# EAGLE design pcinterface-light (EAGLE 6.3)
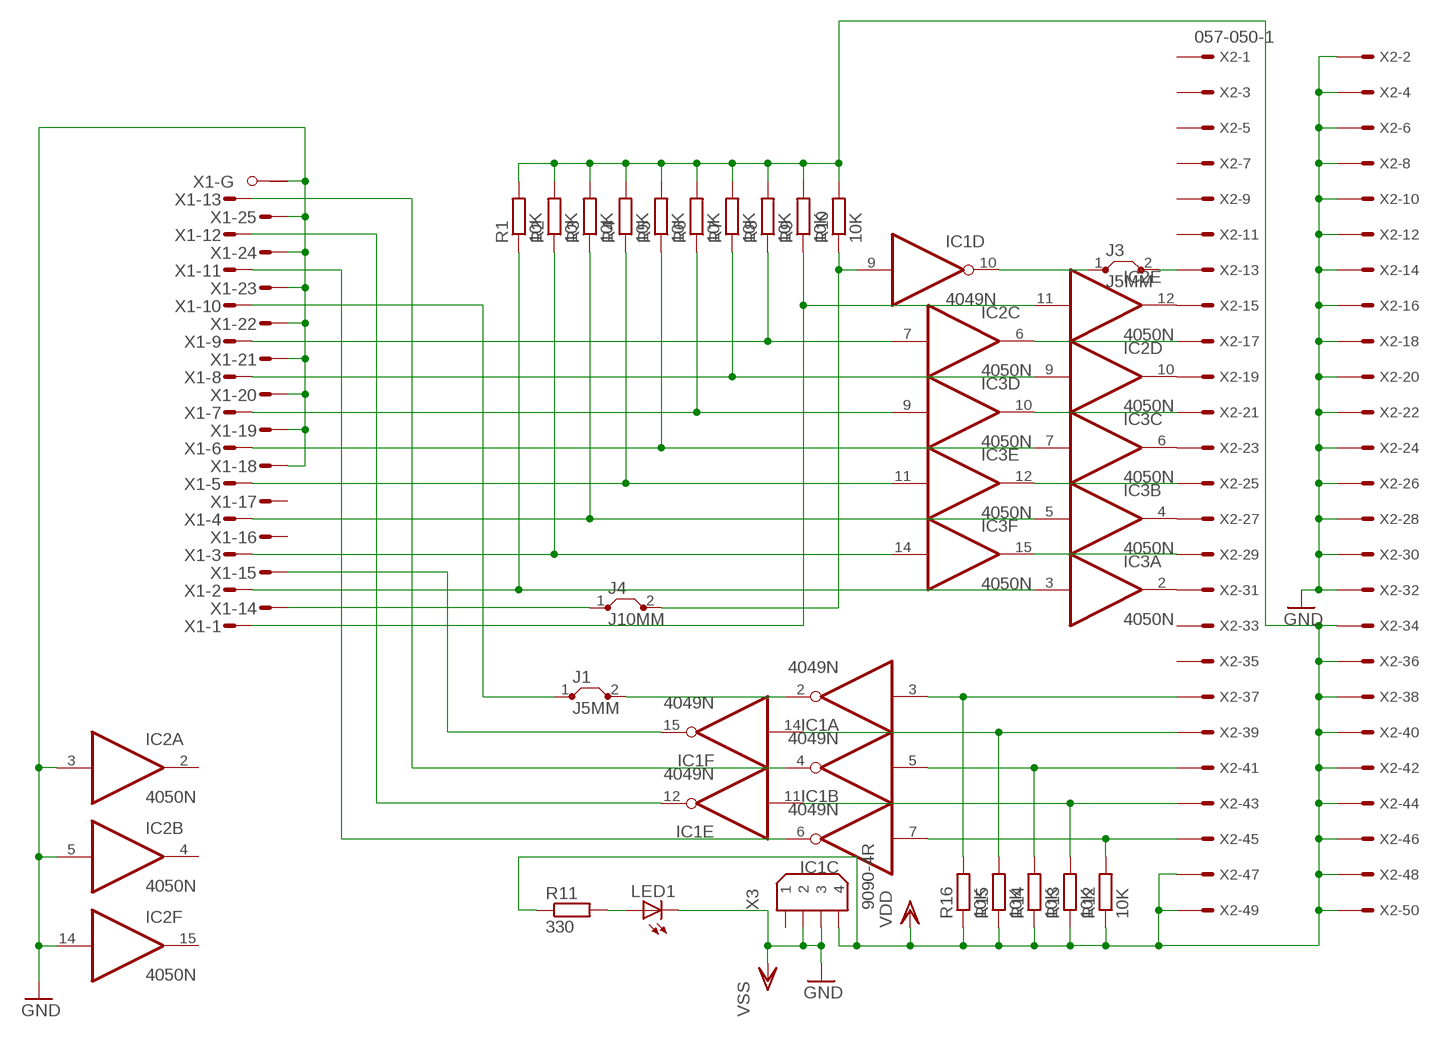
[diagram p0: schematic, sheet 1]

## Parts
IC1  4049N  [DIL16]
IC2  4050N  [DIL16]
IC3  4050N  [DIL16]
J1  J5MM  [05]
J3  J5MM  [05]
J4  J10MM  [10]
LED1  LED3MM  [LED3MM]
R1  10K  R-EU_0207/10  [0207/10]
R2  10K  R-EU_0207/10  [0207/10]
R3  10K  R-EU_0207/10  [0207/10]
R4  10K  R-EU_0207/10  [0207/10]
R5  10K  R-EU_0207/10  [0207/10]
R6  10K  R-EU_0207/10  [0207/10]
R7  10K  R-EU_0207/10  [0207/10]
R8  10K  R-EU_0207/10  [0207/10]
R9  10K  R-EU_0207/10  [0207/10]
R10  10K  R-EU_0207/10  [0207/10]
R11  330  R-EU_0207/10  [0207/10]
R12  10K  R-EU_0207/10  [0207/10]
R13  10K  R-EU_0207/10  [0207/10]
R14  10K  R-EU_0207/10  [0207/10]
R15  10K  R-EU_0207/10  [0207/10]
R16  10K  R-EU_0207/10  [0207/10]
X1  M25HPS  [M25HP]
X2  057-050-1  [057-050-1]
X3  9090-4R  [9090-4R]

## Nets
N$1: J4.1 X1.14(-14:M)
N$2: LED1.A R11.2
N$3: IC2.12(E:O) X2.15
N$4: IC2.6(C:O) X2.17
N$5: IC2.10(D:O) X2.19
N$6: IC3.10(D:O) X2.21
N$7: IC3.6(C:O) X2.23
N$8: IC3.12(E:O) X2.25
N$9: IC3.4(B:O) X2.27
N$10: IC3.15(F:O) X2.29
N$11: IC3.2(A:O) X2.31
N$12: IC1.9(D:I) J4.2 R10.1
N$13: IC2.11(E:I) R9.1 X1.1(-1:M)
N$14: IC2.7(C:I) R8.1 X1.9(-9:M)
N$15: IC2.9(D:I) R7.1 X1.8(-8:M)
N$16: IC3.9(D:I) R6.1 X1.7(-7:M)
N$17: IC3.7(C:I) R5.1 X1.6(-6:M)
N$18: IC3.11(E:I) R4.1 X1.5(-5:M)
N$19: IC3.5(B:I) R3.1 X1.4(-4:M)
N$20: IC3.14(F:I) R2.1 X1.3(-3:M)
N$21: IC3.3(A:I) R1.1 X1.2(-2:M)
N$22: IC1.7(C:I) R12.2 X2.45
N$23: IC1.11(E:I) R13.2 X2.43
N$24: IC1.5(B:I) R14.2 X2.41
N$25: IC1.14(F:I) R15.2 X2.39
N$26: IC1.3(A:I) R16.2 X2.37
N$28: IC1.6(C:O) X1.11(-11:M)
N$29: IC1.12(E:O) X1.12(-12:M)
N$30: IC1.4(B:O) X1.13(-13:M)
N$31: IC1.15(F:O) X1.15(-15:M)
N$32: J1.1 X1.10(-10:M)
N$34: IC1.2(A:O) J1.2
N$35: IC1.10(D:O) J3.1
N$36: J3.2 X2.13
VDD: R1.2 R2.2 R3.2 R4.2 R5.2 R6.2 R7.2 R8.2 R9.2 R10.2 R11.1 R12.1 R13.1 R14.1 R15.1 R16.1 X2.34 X2.36 X2.38 X2.40 X2.42 X2.44 X2.46 X2.47 X2.48 X2.49 X2.50 X3.4
VSS: IC2.3(A:I) IC2.5(B:I) IC2.14(F:I) LED1.K(C) X1.18(-18:M) X1.19(-19:M) X1.20(-20:M) X1.21(-21:M) X1.22(-22:M) X1.23(-23:M) X1.24(-24:M) X1.25(-25:M) X1.G1(-G:G1) X2.2 X2.4 X2.6 X2.8 X2.10 X2.12 X2.14 X2.16 X2.18 X2.20 X2.22 X2.24 X2.26 X2.28 X2.30 X2.32 X3.2 X3.3 ; supply symbol labelled GND
Unconnected: IC2.2(A:O) IC2.4(B:O) IC2.15(F:O) X1.16(-16:M) X1.17(-17:M) X1.G2(-G:G2) X2.1 X2.3 X2.5 X2.7 X2.9 X2.11 X2.33 X2.35 X3.1

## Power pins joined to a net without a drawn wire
VDD: IC1.1(P:VDD) IC2.1(P:VDD) IC3.1(P:VDD)
VSS: IC1.8(P:VSS) IC2.8(P:VSS) IC3.8(P:VSS)

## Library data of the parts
IC1 = 40xx:4049: Hex inverting BUFFER
IC2 IC3 = 40xx:4050: Hex non-inverting BUFFER
J1 J3 J4 = jumper:J: Bridge
LED1 = led:LED: LED
R1-R16 = resistor:R-EU_: RESISTOR, European symbol
X1 = con-subd:M25HPS: SUB-D; OC_FARNELL: unknown; OC_NEWARK: unknown
X2 = con-panduit:057-050-: CONNECTOR 50-pin series 057 contact pc board low profile headers; OC_FARNELL: unknown; OC_NEWARK: unknown
X3 = con-thomas-betts:9090-4: Disk Drive Power four position Source: Thomas & Betts Electronic Interconnects Eiropean Edition 1998; OC_FARNELL: unknown; OC_NEWARK: unknown

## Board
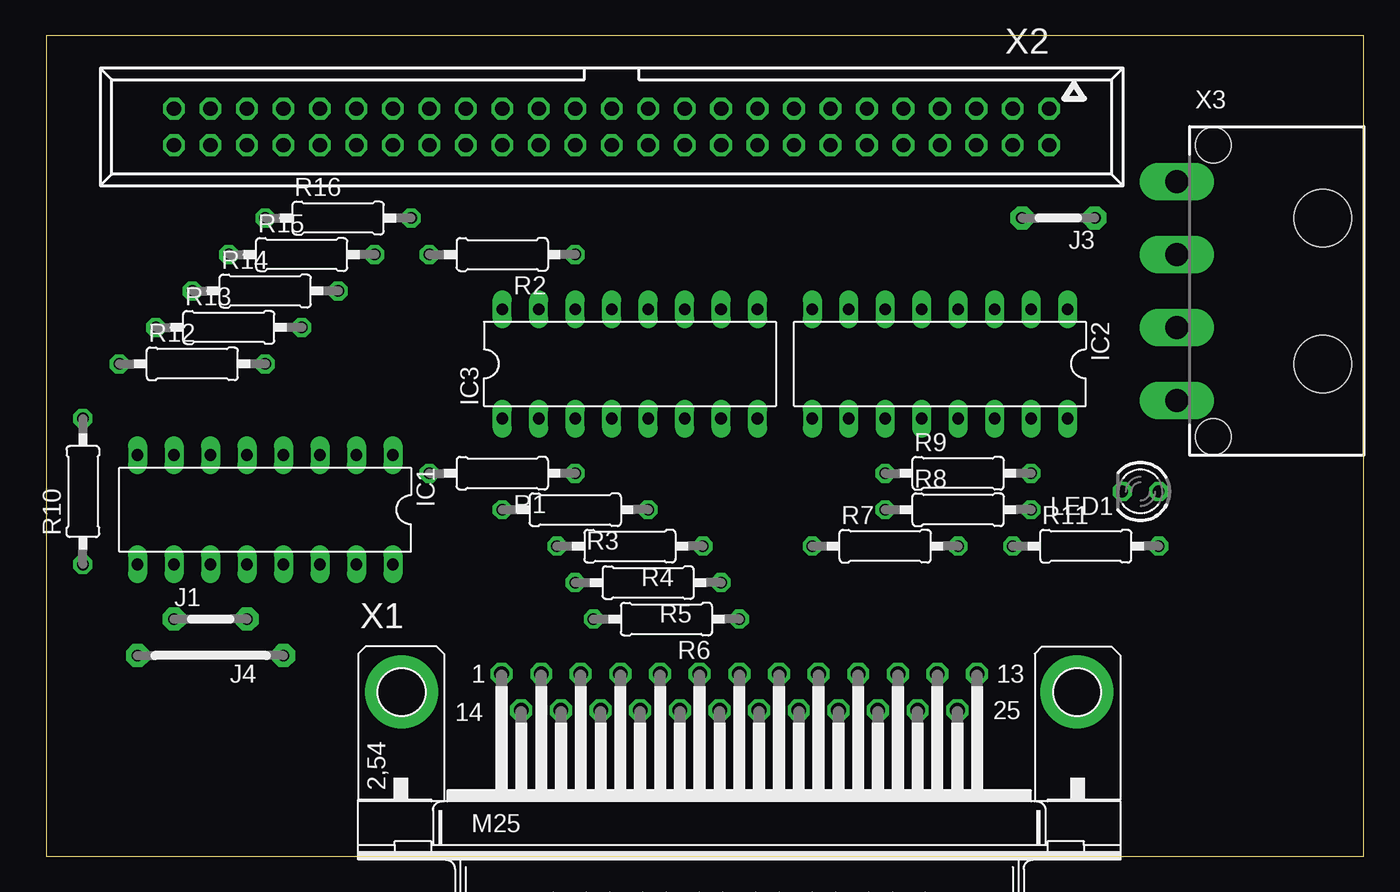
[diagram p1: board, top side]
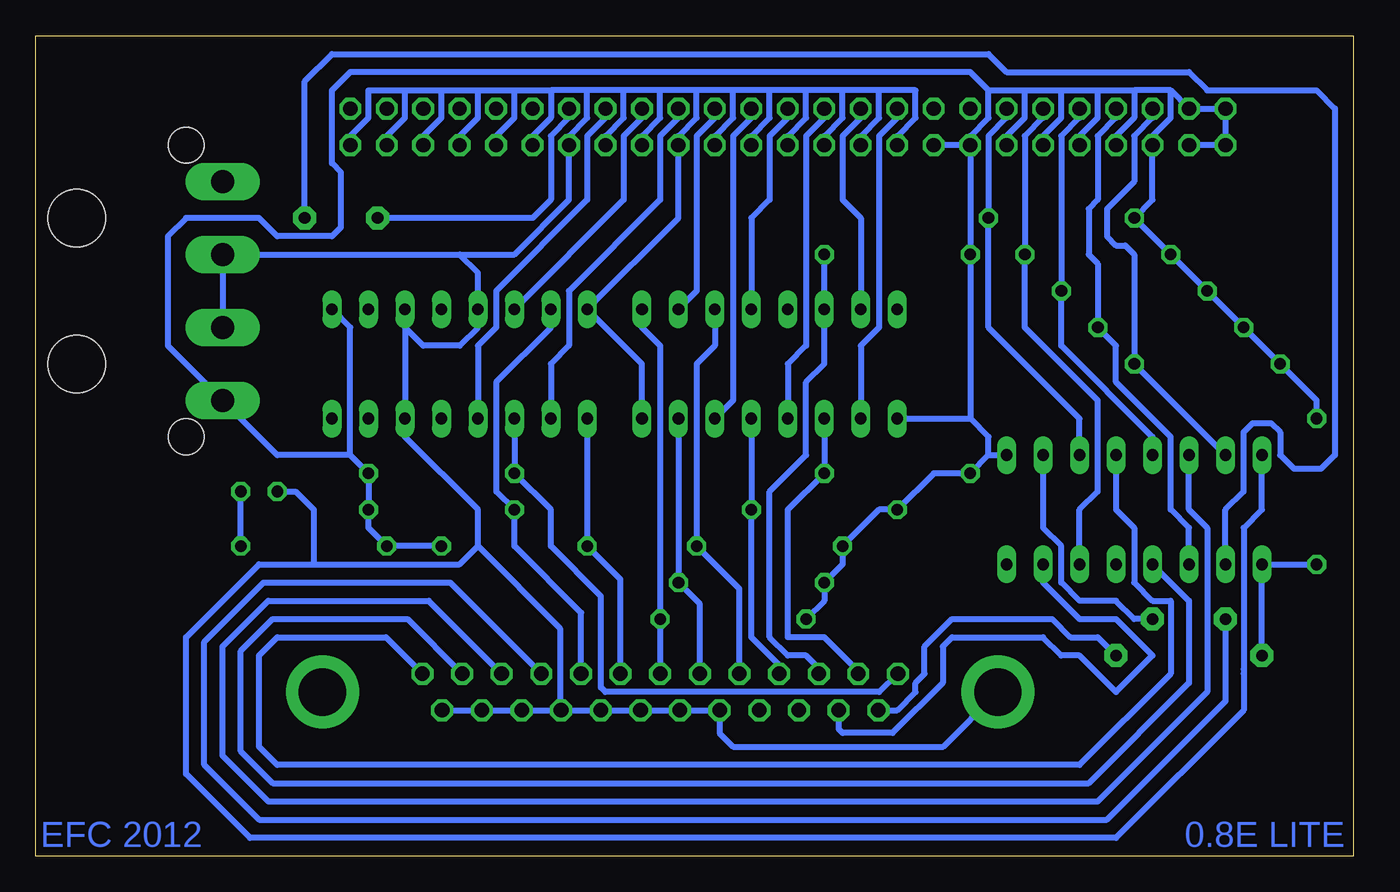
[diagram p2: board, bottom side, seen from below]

Size 91.75 x 57.14 mm. Coordinates in mm from the lower left corner, seen from the top.
Outline: 0,0 91.75,0 91.75,57.14 0,57.14 0,0
Copper layers (1*16): Top 0.035mm / dielectric 1.5mm / Bottom 0.035mm
Design rules "default": minimum track width 10mil, minimum drill 24mil, track to track 8mil, track to pad 8mil, pad to pad 8mil, via to via 8mil, smd to smd 8mil, copper to edge 40mil, drill to drill 8mil, minimum pad ring 10mil, minimum via ring 8mil, stop-mask expansion 4mil, vias tented up to drill 0mil, thermal gap 10mil

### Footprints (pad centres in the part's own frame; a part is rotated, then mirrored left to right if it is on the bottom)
DIL16 = drill 0.813 long: 1 -8.89,-3.81; 2 -6.35,-3.81; 3 -3.81,-3.81; 4 -1.27,-3.81; 5 1.27,-3.81; 6 3.81,-3.81; 7 6.35,-3.81; 8 8.89,-3.81; 9 8.89,3.81; 10 6.35,3.81; 11 3.81,3.81; 12 1.27,3.81; 13 -1.27,3.81; 14 -3.81,3.81; 15 -6.35,3.81; 16 -8.89,3.81
05 = drill 0.813 pad 1.6 octagon: 1 -2.54,0; 2 2.54,0
10 = drill 0.813 pad 1.6 octagon: 1 -5.08,0; 2 5.08,0
LED3MM = drill 0.813 octagon: A -1.27,0; K 1.27,0
0207/10 = drill 0.813 octagon: 1 -5.08,0; 2 5.08,0
M25HP = drill 1.016 octagon: 1 -16.561,1.27; 2 -13.792,1.27; 3 -11.049,1.27; 4 -8.28,1.27; 5 -5.512,1.27; 6 -2.769,1.27; 7 0,1.27; 8 2.769,1.27; 9 5.512,1.27; 10 8.28,1.27; 11 11.049,1.27; 12 13.792,1.27; 13 16.561,1.27; 14 -15.189,-1.27; 15 -12.421,-1.27; 16 -9.652,-1.27; 17 -6.909,-1.27; 18 -4.14,-1.27; 19 -1.372,-1.27; 20 1.372,-1.27; 21 4.14,-1.27; 22 6.909,-1.27; 23 9.652,-1.27; 24 12.421,-1.27; 25 15.189,-1.27 | drill 3.302 pad 5.08: G1 -23.52,0; G2 23.52,0
057-050-1 = drill 1 octagon: 1 -30.48,-1.27; 2 -30.48,1.27; 3 -27.94,-1.27; 4 -27.94,1.27; 5 -25.4,-1.27; 6 -25.4,1.27; 7 -22.86,-1.27; 8 -22.86,1.27; 9 -20.32,-1.27; 10 -20.32,1.27; 11 -17.78,-1.27; 12 -17.78,1.27; 13 -15.24,-1.27; 14 -15.24,1.27; 15 -12.7,-1.27; 16 -12.7,1.27; 17 -10.16,-1.27; 18 -10.16,1.27; 19 -7.62,-1.27; 20 -7.62,1.27; 21 -5.08,-1.27; 22 -5.08,1.27; 23 -2.54,-1.27; 24 -2.54,1.27; 25 0,-1.27; 26 0,1.27; 27 2.54,-1.27; 28 2.54,1.27; 29 5.08,-1.27; 30 5.08,1.27; 31 7.62,-1.27; 32 7.62,1.27; 33 10.16,-1.27; 34 10.16,1.27; 35 12.7,-1.27; 36 12.7,1.27; 37 15.24,-1.27; 38 15.24,1.27; 39 17.78,-1.27; 40 17.78,1.27; 41 20.32,-1.27; 42 20.32,1.27; 43 22.86,-1.27; 44 22.86,1.27; 45 25.4,-1.27; 46 25.4,1.27; 47 27.94,-1.27; 48 27.94,1.27; 49 30.48,-1.27; 50 30.48,1.27
9090-4R = drill 1.6 pad 2.6 long: 1 -7.62,-6.35; 2 -2.54,-6.35; 3 2.54,-6.35; 4 7.62,-6.35 | hole 4: -5.08,3.81; 5.08,3.81 | hole 2.5: -10.16,-3.81; 10.16,-3.81

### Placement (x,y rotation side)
IC1  15.24,24.13 180 top
IC2  62.23,34.29 180 top
IC3  40.64,34.29 0 top
J1  11.43,16.51 0 top
J3  70.48,44.45 180 top
J4  11.43,13.97 180 top
LED1  76.2,25.4 180 top
R1  31.75,26.67 180 top
R2  31.75,41.91 180 top
R3  36.83,24.13 180 top
R4  40.64,21.59 180 top
R5  41.91,19.05 180 top
R6  43.18,16.51 180 top
R7  58.42,21.59 0 top
R8  63.5,24.13 0 top
R9  63.5,26.67 0 top
R10  2.54,25.4 90 top
R11  72.39,21.59 0 top
R12  10.16,34.29 0 top
R13  12.7,36.83 0 top
R14  15.24,39.37 0 top
R15  17.78,41.91 0 top
R16  20.32,44.45 0 top
X1  48.26,11.43 0 top
X2  39.37,50.8 180 top
X3  85.09,39.37 270 top

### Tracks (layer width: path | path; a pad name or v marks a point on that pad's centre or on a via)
N$1
  Bottom 0.406: X1.14 31.75,10.16 30.48,11.43 30.48,12.06 29.84,12.7 29.84,14.61 27.94,16.51 20.95,16.51 19.69,15.24 17.78,15.24 J4.1
N$2
  Bottom 0.406: R11.2 LED1.A
N$3
  Bottom 0.406: X2.15 52.07,51.44 53.34,50.17 53.34,45.72 59.69,39.37 59.69,36.83 60.96,35.56 IC2.12
N$4
  Bottom 0.406: X2.17 49.53,51.44 50.8,50.17 50.8,45.72 IC2.6
N$5
  Bottom 0.406: X2.19 46.99,51.44 48.26,50.17 48.26,45.72 54.61,39.37 54.61,35.56 55.88,34.29 IC2.10
N$6
  Bottom 0.406: X2.21 44.45,51.44 45.72,50.17 45.72,39.37 IC3.10
N$7
  Bottom 0.406: X2.23 41.91,51.44 43.18,50.17 43.18,31.75 IC3.6
N$8
  Bottom 0.406: X2.25 39.37,51.44 40.64,50.17 40.64,45.72 41.91,44.45 IC3.12
N$9
  Bottom 0.406: X2.27 36.83,51.44 38.1,50.17 38.1,35.56 39.37,34.29 IC3.4
N$10
  Bottom 0.406: X2.29 34.29,51.44 35.56,50.17 35.56,45.72 34.29,44.45 IC3.15
N$11
  Bottom 0.406: X2.31 31.75,51.44 33.02,50.17 33.02,36.83 34.29,35.56 IC3.2
N$12
  Bottom 0.406: R10.1 IC1.9 J4.2
N$13
  Bottom 0.406: IC2.11 R9.1 55.88,24.13 55.88,21.59 52.39,18.1 52.39,11.75 52.07,11.43 33.02,11.43 31.75,12.7 X1.1
N$14
  Bottom 0.406: IC2.7 55.88,36.83 59.69,33.02 59.69,25.4 R8.1 58.42,21.59 53.77,16.94 X1.9
N$15
  Bottom 0.406: IC2.9 R7.1 51.03,19.28 X1.8
N$16
  Bottom 0.406: IC3.9 49.53,36.83 48.26,35.56 R6.1 X1.7
N$17
  Bottom 0.406: IC3.7 R5.1 45.49,17.55 X1.6
N$18
  Bottom 0.406: IC3.11 44.45,35.56 45.72,34.29 R4.1 42.75,18.62 X1.5
N$19
  Bottom 0.406: IC3.5 R3.1 41.91,15.24 39.98,13.31 X1.4
N$20
  Bottom 0.406: R2.1 IC3.14 36.83,34.29 38.1,33.02 38.1,27.94 40.64,25.4 40.64,15.24 39.37,13.97 38.1,13.97 37.21,13.08 X1.3
N$21
  Bottom 0.406: IC3.3 R1.1 39.37,24.13 39.37,15.24 36.83,15.24 34.47,12.88 X1.2
N$22
  Bottom 0.406: X2.45 13.97,51.44 15.24,50.17 15.24,46.99 17.15,45.08 17.15,43.18 16.51,42.55 15.87,42.55 15.24,41.91 R12.2 IC1.7
N$23
  Bottom 0.406: X2.43 16.51,51.44 17.78,50.17 17.78,45.72 18.41,45.08 18.41,41.91 17.78,41.28 R13.2 16.51,35.56 16.51,33.02 12.7,29.21 12.7,24.13 11.43,22.86 IC1.11
N$24
  Bottom 0.406: X2.41 19.05,51.44 20.32,50.17 R14.2 20.32,35.56 13.97,29.21 IC1.5
N$25
  Bottom 0.406: X2.39 21.59,51.44 22.86,50.17 R15.2 22.86,36.83 17.78,31.75 17.78,25.4 19.05,24.13 IC1.14
N$26
  Bottom 0.406: X2.37 24.13,51.44 25.4,50.17 R16.2 25.4,36.83 19.05,30.48 IC1.3
N$28
  Bottom 0.406: X1.11 64.39,17.78 75.56,17.78 78.74,14.61 78.74,6.98 75.56,3.81 17.78,3.81 10.16,11.43 10.16,22.86 11.43,24.13 IC1.6
N$29
  Bottom 0.406: X1.12 65.86,16.51 75.25,16.51 77.47,14.29 77.47,7.3 75.25,5.08 18.41,5.08 11.43,12.06 11.43,17.78 IC1.12
N$30
  Bottom 0.406: 64.82,12.75 X1.13 67.36,15.24 74.93,15.24 76.2,13.97 76.2,7.62 74.93,6.35 19.05,6.35 12.7,12.7 12.7,17.78 13.97,17.78 15.24,19.05 15.24,22.86 16.51,24.13 IC1.4
N$31
  Bottom 0.406: X1.15 35.84,8.85 35.56,8.57 32.07,8.57 28.58,12.06 28.58,14.61 27.94,15.24 21.59,15.24 20.32,13.97 19.05,13.97 16.51,11.43 13.97,13.97 16.51,16.51 19.05,16.51 21.59,19.05 IC1.15
N$32
  Bottom 0.406: X1.10 62.89,19.05 75.88,19.05 80.01,14.92 80.01,6.35 76.2,2.54 17.15,2.54 8.89,10.8 J1.1
N$34
  Bottom 0.406: IC1.2 21.59,22.86 20.32,21.59 20.32,19.05 19.05,17.78 16.51,17.78 15.24,16.51 J1.2
N$35
  Bottom 0.406: IC1.10 8.89,24.13 7.62,25.4 7.62,29.53 6.98,30.16 5.71,30.16 5.08,29.53 5.08,27.94 4.13,26.99 2.22,26.99 1.27,27.94 1.27,52.07 2.54,53.34 10.16,53.34 11.43,54.61 24.13,54.61 25.4,55.88 71.12,55.88 73.03,53.97 J3.1
N$36
  Bottom 0.406: X2.13 54.61,51.44 55.88,50.17 55.88,45.72 57.15,44.45 J3.2
VDD
  Bottom 0.406: 26.67,30.48 R2.2 X2.36 | 12.7,53.34 12.7,51.44 13.97,50.17 X2.46 13.97,45.72 R16.1 R15.1 R14.1 R13.1 R12.1 2.54,31.75 R10.2 | 12.7,53.34 15.24,53.34 | 15.24,53.34 15.24,51.44 16.51,50.17 X2.44 | X2.42 19.05,50.17 17.78,51.44 17.78,53.34 | 17.78,53.34 15.24,53.34 | X2.40 21.59,50.17 20.32,51.44 20.32,53.34 | 20.32,53.34 17.78,53.34 | X2.38 24.13,50.17 22.86,51.44 22.86,53.34 | 22.86,53.34 20.32,53.34 | X2.36 26.67,50.17 25.4,51.44 25.4,53.34 | 25.4,53.34 22.86,53.34 | X2.36 X2.34 | 12.7,53.34 X2.47 X2.49 X2.50 X2.48 | 25.4,53.34 26.67,54.61 69.85,54.61 71.12,53.34 71.12,48.26 70.48,47.62 70.48,43.81 71.12,43.18 74.93,43.18 76.2,44.45 81.28,44.45 82.55,43.18 82.55,35.56 X3.4 74.93,27.94 69.85,27.94 | IC3.1 26.67,30.48 | R6.2 36.83,17.78 R5.2 35.56,20.32 R4.2 33.02,24.13 R3.2 29.21,26.67 R1.2 25.4,27.94 | 69.85,27.94 69.85,36.83 IC2.1 | 25.4,27.94 25.4,29.21 26.67,30.48 | 25.4,27.94 IC1.1 | R7.2 R11.1 68.58,22.86 R8.2 R9.2 69.85,27.94
VSS
  Bottom 0.406: X2.12 57.15,50.17 55.88,51.44 55.88,53.34 | 53.34,53.34 53.34,51.44 54.61,50.17 X2.14 54.61,45.72 58.42,41.91 62.23,41.91 | 53.34,53.34 55.88,53.34 | X2.10 59.69,50.17 58.42,51.44 58.42,53.34 | 58.42,53.34 55.88,53.34 | X2.8 62.23,50.17 60.96,51.44 60.96,53.34 | 60.96,53.34 58.42,53.34 | X2.6 64.77,50.17 63.5,51.44 63.5,53.34 | 63.5,53.34 60.96,53.34 | X2.4 67.31,50.17 66.04,51.44 66.04,53.34 | 66.04,53.34 63.5,53.34 | X2.2 69.85,50.17 68.58,51.44 68.58,53.34 66.04,53.34 | X2.16 52.07,50.17 50.8,51.44 50.8,53.34 | 50.8,53.34 53.34,53.34 | X2.18 49.53,50.17 48.26,51.44 48.26,53.34 | 48.26,53.34 50.8,53.34 | 45.72,53.34 45.72,51.44 46.99,50.17 X2.20 46.99,44.45 IC2.8 49.53,34.29 IC3.8 | 45.72,53.34 48.26,53.34 | X2.22 44.45,50.17 43.18,51.44 43.18,53.34 | 43.18,53.34 45.72,53.34 | X2.24 41.91,50.17 40.64,51.44 40.64,53.34 | 40.64,53.34 43.18,53.34 | X2.26 39.37,50.17 38.1,51.44 38.1,53.34 | 38.1,53.34 40.64,53.34 | X2.28 36.83,50.17 35.56,51.44 35.56,53.34 | 35.56,53.34 38.1,53.34 | X2.30 34.29,50.17 33.02,51.44 33.02,53.34 | 33.02,53.34 35.56,53.34 | X2.32 31.75,50.17 30.48,51.44 30.48,53.34 33.02,53.34 | X3.3 X3.2 62.23,41.91 | X1.25 X1.24 X1.23 X1.22 | X1.22 X1.21 X1.20 X1.19 X1.18 44.12,8.56 43.18,7.62 28.55,7.62 X1.G1 | X1.22 55.25,10.24 55.25,15.88 60.96,21.59 | 60.96,21.59 60.96,24.13 66.04,29.21 IC2.14 IC2.3 66.04,36.83 64.77,35.56 62.23,35.56 60.96,36.83 IC2.5 60.96,40.64 62.23,41.91 | 72.39,20.32 76.2,20.32 81.28,15.24 81.28,5.71 76.84,1.27 16.51,1.27 7.62,10.16 7.62,12.7 7.62,13.02 7.62,22.86 6.35,24.13 IC1.8 | 72.39,20.32 62.23,20.32 60.96,21.59 | LED1.K 73.66,25.4 72.39,24.13 72.39,20.32

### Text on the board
Bottom: 0.8E LITE | EFC 2012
